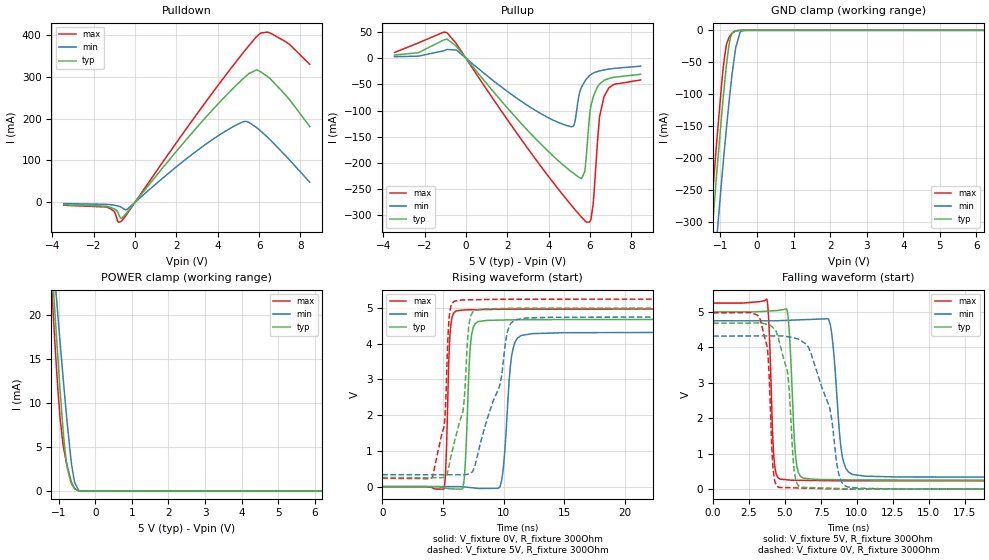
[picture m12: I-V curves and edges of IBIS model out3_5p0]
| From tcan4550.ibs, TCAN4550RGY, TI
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|   out3_5p0 Model
[Model]   out3_5p0
Model_type   3-state
Polarity   Non-Inverting
Vmeas = 2.5
Vref = 0
Cref = 2pF
Rref = 100000
|   typ   min   max
C_comp   6.133pF   5.723pF   6.333pF
|  Where Nom  PVT is Nominal Process, 5V, 27C
|   Fast PVT is Strong Process,  5.25, -40C
|   Slow PVT is Weak Process,   4.75V, 150C
[Voltage Range]   5   4.75   5.25
|Junction Temperature
[Temperature Range]   27   150   -40
[Pullup Reference]   5   4.75   5.25
[Pulldown Reference]   0   0   0
[Power Clamp Reference]   5   4.75   5.25
[GND Clamp Reference]   0   0   0
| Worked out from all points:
|   slope of the pulldown table from 0 to 0.75 V, typ, clamps not added: 16.1 ohm
|   slope of the pullup table from 0 to 0.75 V, typ, clamps not added: 20.6 ohm
|   GND clamp passes 1 mA (typ) near -0.59 V on its own axis
|   POWER clamp passes 1 mA (typ) near -0.67 V on its own axis
|   falling waveform, V_fixture 5V, R_fixture 300Ohm: 20-80 % time 327ps typ, 496ps min, 252ps max; typ from 5 V to 0.254 V
|   rising waveform, V_fixture 0V, R_fixture 300Ohm: 20-80 % time 337ps typ, 523ps min, 252ps max; typ from 0 V to 4.68 V
|   rising waveform, V_fixture 5V, R_fixture 300Ohm: 20-80 % time 1.11ns typ, 2ns min, 668ps max; typ from 0.254 V to 5 V
|   falling waveform, V_fixture 0V, R_fixture 300Ohm: 20-80 % time 686ps typ, 1.45ns min, 339ps max; typ from 4.68 V to 0 V
[Pulldown]
|   Voltage   I(typ)   I(min)   I(max)
-3.45V    -6.027mA   -3.203mA   -7.208mA
-1.391V   -9.389mA   -4.966mA   -11.46mA
-1.01V    -15.55mA   -7.076mA   -21.61mA
-796.3mV  -27.51mA   -9.375mA   -47.58mA
-641.6mV  -38.29mA   -12.53mA   -44.32mA
-415.5mV  -25.93mA   -17.69mA   -30mA
4.535V    262mA      174.7mA    313.5mA
5.285V    298mA      193.2mA    360.9mA
5.88V     316.2mA    178.5mA    396.2mA
6.558V    294.2mA    148.2mA    404mA
7.474V    245mA      100.9mA    377.2mA
8.45V     180.9mA    47.81mA    329.8mA
[GND Clamp]
|   Voltage   I(typ)   I(min)   I(max)
-3.45V    -2.161A    -2.181A    -2.165A
-1.379V   -435mA     -529.9mA   -389.2mA
-1.225V   -315.3mA   -414.9mA   -266.8mA
-1.213V   -306.4mA   -406.3mA   -257.7mA
-1.094V   -219.6mA   -321.4mA   -169.8mA
-939.1mV  -115.9mA   -217.7mA   -67.9mA
-843.9mV  -59.69mA   -158.8mA   -24.88mA
-724.9mV  -11.58mA   -91.52mA   -7.504mA
-582.1mV  -603.2uA   -27.32mA   -743.2uA
-463.1mV  -32.89uA   -3.456mA   -28.75uA
-320.3mV  -324.9nA   -97.95uA   -6.312nA
8.45V     0A         0A         0A
[Pullup]
|   Voltage   I(typ)   I(min)   I(max)
-3.45V    5.973mA    2.768mA    10.82mA
-915.3mV  36.43mA    16.52mA    48.62mA
5.035V    -214.4mA   -130.2mA   -277.3mA
5.261V    -221.3mA   -123.6mA   -288mA
5.594V    -229.7mA   -55.31mA   -303.3mA
5.808V    -194.5mA   -40.87mA   -312.3mA
6.046V    -91.25mA   -31.19mA   -307.7mA
6.153V    -74.62mA   -28.65mA   -279.2mA
6.463V    -49.46mA   -24.29mA   -112mA
6.689V    -42.32mA   -22.35mA   -72.71mA
7.153V    -36.51mA   -19.58mA   -50.05mA
8.45V     -30.72mA   -15.21mA   -41.54mA
[POWER Clamp]
|   Voltage   I(typ)   I(min)   I(max)
-3.45V    188.5mA    154.1mA    200.6mA
-1.344V   36.46mA    36.78mA    34.14mA
-1.094V   19.64mA    23.61mA    16.1mA
-1.07V    18.11mA    22.38mA    14.52mA
-1.058V   17.35mA    21.77mA    13.75mA
-962.9mV  11.49mA    16.95mA    8.294mA
-867.7mV  6.319mA    12.3mA     4.954mA
-784.4mV  3.084mA    8.436mA    3.145mA
-641.6mV  746.5uA    2.819mA    899.6uA
-570.2mV  256.9uA    1.035mA    286.9uA
-463.1mV  24.15uA    111uA      17.8uA
8.45V     0A         0A         0A
[Ramp]
R_load = 300
|   typ   min   max
dV/dt_r   2.80884/3.33757e-10   2.59075/5.18927e-10   2.98374/2.51642e-10
dV/dt_f   2.84781/3.25507e-10   2.64923/4.93747e-10   3.01104/2.51548e-10
[Falling Waveform]
V_fixture = 5V
V_fixture_min = 4.75V
V_fixture_max = 5.25V
R_fixture = 300Ohm
C_fixture = 0F
|   Time   V(typ)   V(min)   V(max)
0s        5V         4.75V      5.25V
3.748ns   5.022V     4.749V     5.345V
4.219ns   5.033V     4.749V     945.6mV
4.646ns   5.051V     4.755V     284.6mV
5.204ns   4.897V     4.764V     261.9mV
5.731ns   948.7mV    4.772V     250.3mV
6.243ns   315.7mV    4.78V      247.8mV
8.039ns   270.5mV    4.789V     239.1mV
9.667ns   260.5mV    419.6mV    236.1mV
30ns      253.7mV    334.6mV    231.6mV
[Rising Waveform]
V_fixture = 0V
V_fixture_min = 0V
V_fixture_max = 0V
R_fixture = 300Ohm
C_fixture = 0F
|   Time   V(typ)   V(min)   V(max)
0s        925nV      8.691uV    178.3nV
5.076ns   -31.36mV   177uV      -72.08mV
5.587ns   -63.23mV   193.9uV    4.263V
6.07ns    -67.54mV   210uV      4.914V
6.724ns   119.1mV    -9.575mV   4.944V
7.278ns   3.99V      -28.04mV   4.95V
7.866ns   4.614V     -47.62mV   4.954V
9.729ns   4.661V     22.9mV     4.965V
11.44ns   4.674V     4.225V     4.969V
30ns      4.681V     4.318V     4.973V
[Rising Waveform]
V_fixture = 5V
V_fixture_min = 4.75V
V_fixture_max = 5.25V
R_fixture = 300Ohm
C_fixture = 0F
|   Time   V(typ)   V(min)   V(max)
0s        253.7mV    334.6mV    231.6mV
4.155ns   247.7mV    331.5mV    279.4mV
5.108ns   262.8mV    330.8mV    1.726V
5.503ns   588.3mV    330.5mV    4.679V
5.945ns   1.25V      330.2mV    5.191V
6.698ns   2.226V     329.6mV    5.226V
7.059ns   4.224V     347.6mV    5.228V
7.324ns   4.804V     390.8mV    5.23V
10.93ns   4.992V     4.666V     5.246V
30ns      5V         4.75V      5.25V
[Falling Waveform]
|Gnd
V_fixture = 0V
V_fixture_min = 0V
V_fixture_max = 0V
R_fixture = 300Ohm
C_fixture = 0F
|   Time   V(typ)   V(min)   V(max)
0s        4.681V     4.318V     4.973V
3.283ns   4.688V     4.322V     4.788V
3.792ns   4.643V     4.323V     3.911V
4.162ns   4.556V     4.323V     629.7mV
4.564ns   4.221V     4.324V     50.08mV
5.204ns   3.196V     4.3V       42.4mV
5.654ns   488mV      4.264V     37.37mV
6.099ns   54.22mV    4.19V      32.39mV
9.323ns   11.42mV    67.31mV    4.411mV
30ns      925.4nV    8.692uV    179.2nV
